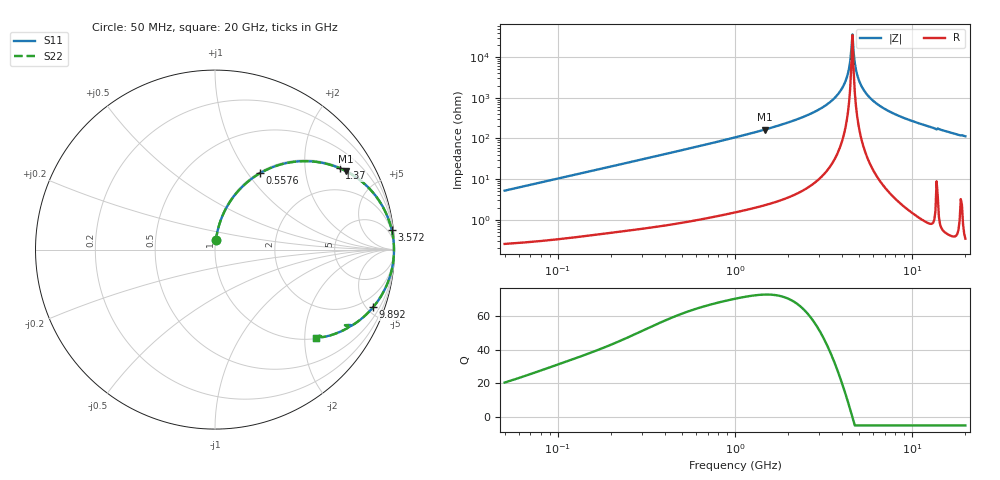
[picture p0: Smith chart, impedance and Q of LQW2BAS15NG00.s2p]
!Murata Part Number: LQW2BAS15NG00
!These Parameters are Measured in Series Mode Connection
!  o--[Z]--o
!Port1  Port2
!  o-------o
!Freq. Start=50[MHz] Stop=20[GHz], 401[Steps]
# Hz S RI R 50
!Freq.(Hz) S11(Real) S11(Imag) S21(Real) S21(Imag) S12(Real) S12(Imag) S22(Real) S22(Imag)
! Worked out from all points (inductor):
!   401 points, 50 MHz to 20 GHz, reference 50 ohm
!   read as one part in series: L = 16.5 nH near 51.52 MHz
!   highest Q = 72.6 at 1.476 GHz (marker M1), where L = 17.9 nH
!   self-resonance near 4.54 GHz
!   S11 on the Smith chart (normalised r, x): 50 MHz: 1.01, +0.10; 557.6 MHz: 1.02, +1.15; 1.37 GHz: 1.04, +3.03; 3.572 GHz: 2, +18; 9.892 GHz: 1.03, -5.48; 20 GHz: 1.01, -2.26
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5e7  0.00522 0.0516  0.9948 -0.0516  0.9948 -0.0516  0.00522 0.0516
1.364002e8  0.023 0.1367  0.977 -0.1367  0.977 -0.1367  0.023 0.1367
3.721004e8  0.1316 0.3292  0.8684 -0.3292  0.8684 -0.3292  0.1316 0.3292
5.575697e8  0.2519 0.4262  0.7481 -0.4262  0.7481 -0.4262  0.2519 0.4262
1e9  0.5296 0.492  0.4704 -0.492  0.4704 -0.492  0.5296 0.492
1.369645e9  0.6947 0.4537  0.3053 -0.4537  0.3053 -0.4537  0.6947 0.4537
1.476162e9  0.7311 0.4366  0.2689 -0.4366  0.2689 -0.4366  0.7311 0.4366
2.728004e9  0.9437 0.2219  0.0563 -0.2219  0.0563 -0.2219  0.9437 0.2219
3.572216e9  0.9849 0.1085  0.0151 -0.1085  0.0151 -0.1085  0.9849 0.1085
3.908127e9  0.9921 0.0701  0.00792 -0.0701  0.00792 -0.0701  0.9921 0.0701
4.149438e9  0.9952 0.0444  0.00483 -0.0444  0.00483 -0.0444  0.9952 0.0444
4.34015e9  0.9966 0.0251  0.00339 -0.0251  0.00339 -0.0251  0.9966 0.0251
4.472136e9  0.9971 0.0122  0.00286 -0.0122  0.00286 -0.0122  0.9971 0.0122
4.608136e9  0.9973 -0.000696  0.00266 0.000696  0.00266 0.000696  0.9973 -0.000696
4.748272e9  0.9972 -0.0136  0.0028 0.0136  0.0028 0.0136  0.9972 -0.0136
4.81993e9  0.997 -0.02  0.003 0.02  0.003 0.02  0.997 -0.02
4.966507e9  0.9964 -0.0329  0.00364 0.0329  0.00364 0.0329  0.9964 -0.0329
5.352748e9  0.9933 -0.0651  0.00672 0.0651  0.00672 0.0651  0.9933 -0.0651
6.125241e9  0.9823 -0.123  0.0177 0.123  0.0177 0.123  0.9823 -0.123
7.442007e9  0.9535 -0.2057  0.0465 0.2057  0.0465 0.2057  0.9535 -0.2057
9.892087e9  0.8812 -0.3208  0.1188 0.3208  0.1188 0.3208  0.8812 -0.3208
2e10  0.5614 -0.4947  0.4386 0.4947  0.4386 0.4947  0.5614 -0.4947
